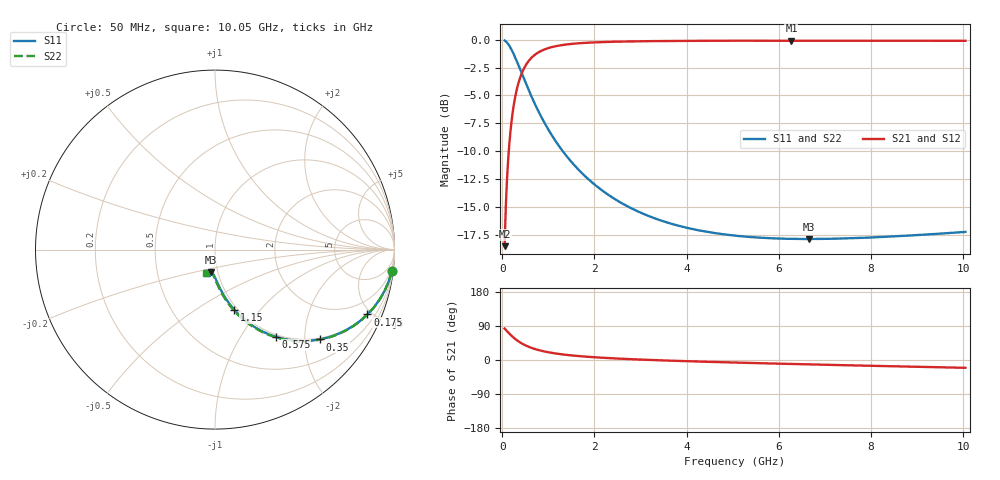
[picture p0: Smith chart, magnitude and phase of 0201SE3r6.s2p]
! AVX Thin Film Operation		Date: August 2001
! Description: Accu-P® Series, Thin Film, SMD, RF Capacitor
! Part Number: 0201YJ3R6ABW
! 50 MHz  -  10.05 GHz
! Serial Measurements
# mhz S db R 50
!	S11		S21		S12		S22
!	dB	Phase	dB	Phase	dB	Phase	dB	Phase
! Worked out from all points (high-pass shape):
!   401 points, 50 MHz to 10.05 GHz, reference 50 ohm
!   highest |S21| = -0.08 dB at 6.275 GHz (marker M1); lowest = -18.5 dB at 50 MHz (marker M2)
!   |S21| within 3 dB of the highest: 416 MHz to end of sweep
!   lowest |S11| = -17.9 dB at 6.65 GHz (marker M3), VSWR 1.29, Z = 46.4 - j11.8 ohm
!   |S11| at or under -10 dB: 1.31 GHz to end of sweep
!   |S22| runs from -17.9 to -0.1 dB; largest |S21 - S12| = 0
!   S11 on the Smith chart (normalised r, x): 50 MHz: 1, -16; 175 MHz: 0.97, -4.72; 350 MHz: 0.97, -2.36; 575 MHz: 0.96, -1.44; 1.15 GHz: 0.96, -0.74; 10.05 GHz: 0.88, -0.23
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50  -0.06 -6.9  -18.54 83.1  -18.54 83.1  -0.06 -6.9
75  -0.14 -10.3  -15.10 79.7  -15.10 79.7  -0.14 -10.4
125  -0.37 -16.9  -10.90 73.1  -10.90 73.1  -0.37 -17.0
175  -0.70 -23.0  -8.31 66.9  -8.31 66.9  -0.70 -23.2
250  -1.32 -31.3  -5.84 58.5  -5.84 58.5  -1.32 -31.5
350  -2.28 -40.6  -3.90 49.3  -3.90 49.3  -2.28 -40.8
450  -3.30 -48.0  -2.75 41.9  -2.75 41.9  -3.30 -48.2
575  -4.55 -55.1  -1.89 34.7  -1.89 34.7  -4.55 -55.4
700  -5.71 -60.5  -1.37 29.2  -1.37 29.2  -5.71 -60.9
825  -6.76 -64.7  -1.04 25.0  -1.04 25.0  -6.76 -65.2
975  -7.90 -68.6  -0.78 21.0  -0.78 21.0  -7.90 -69.2
1150  -9.06 -72.2  -0.58 17.3  -0.58 17.3  -9.06 -72.9
1725  -11.97 -79.7  -0.29 9.7  -0.29 9.7  -11.97 -80.7
2475  -14.40 -85.2  -0.17 3.9  -0.17 3.9  -14.40 -86.5
3400  -16.18 -89.7  -0.12 -0.7  -0.12 -0.7  -16.18 -91.3
4175  -17.05 -92.6  -0.10 -3.8  -0.10 -3.8  -17.05 -94.4
5050  -17.60 -95.4  -0.09 -6.8  -0.09 -6.8  -17.60 -97.4
6275  -17.89 -99.1  -0.08 -10.5  -0.08 -10.5  -17.89 -101.0
6650  -17.90 -100.1  -0.08 -11.6  -0.08 -11.6  -17.90 -102.1
6725  -17.90 -100.3  -0.08 -11.8  -0.08 -11.8  -17.90 -102.3
8400  -17.69 -104.9  -0.08 -16.4  -0.08 -16.4  -17.69 -106.7
10050  -17.26 -109.2  -0.09 -20.6  -0.09 -20.6  -17.27 -110.9
